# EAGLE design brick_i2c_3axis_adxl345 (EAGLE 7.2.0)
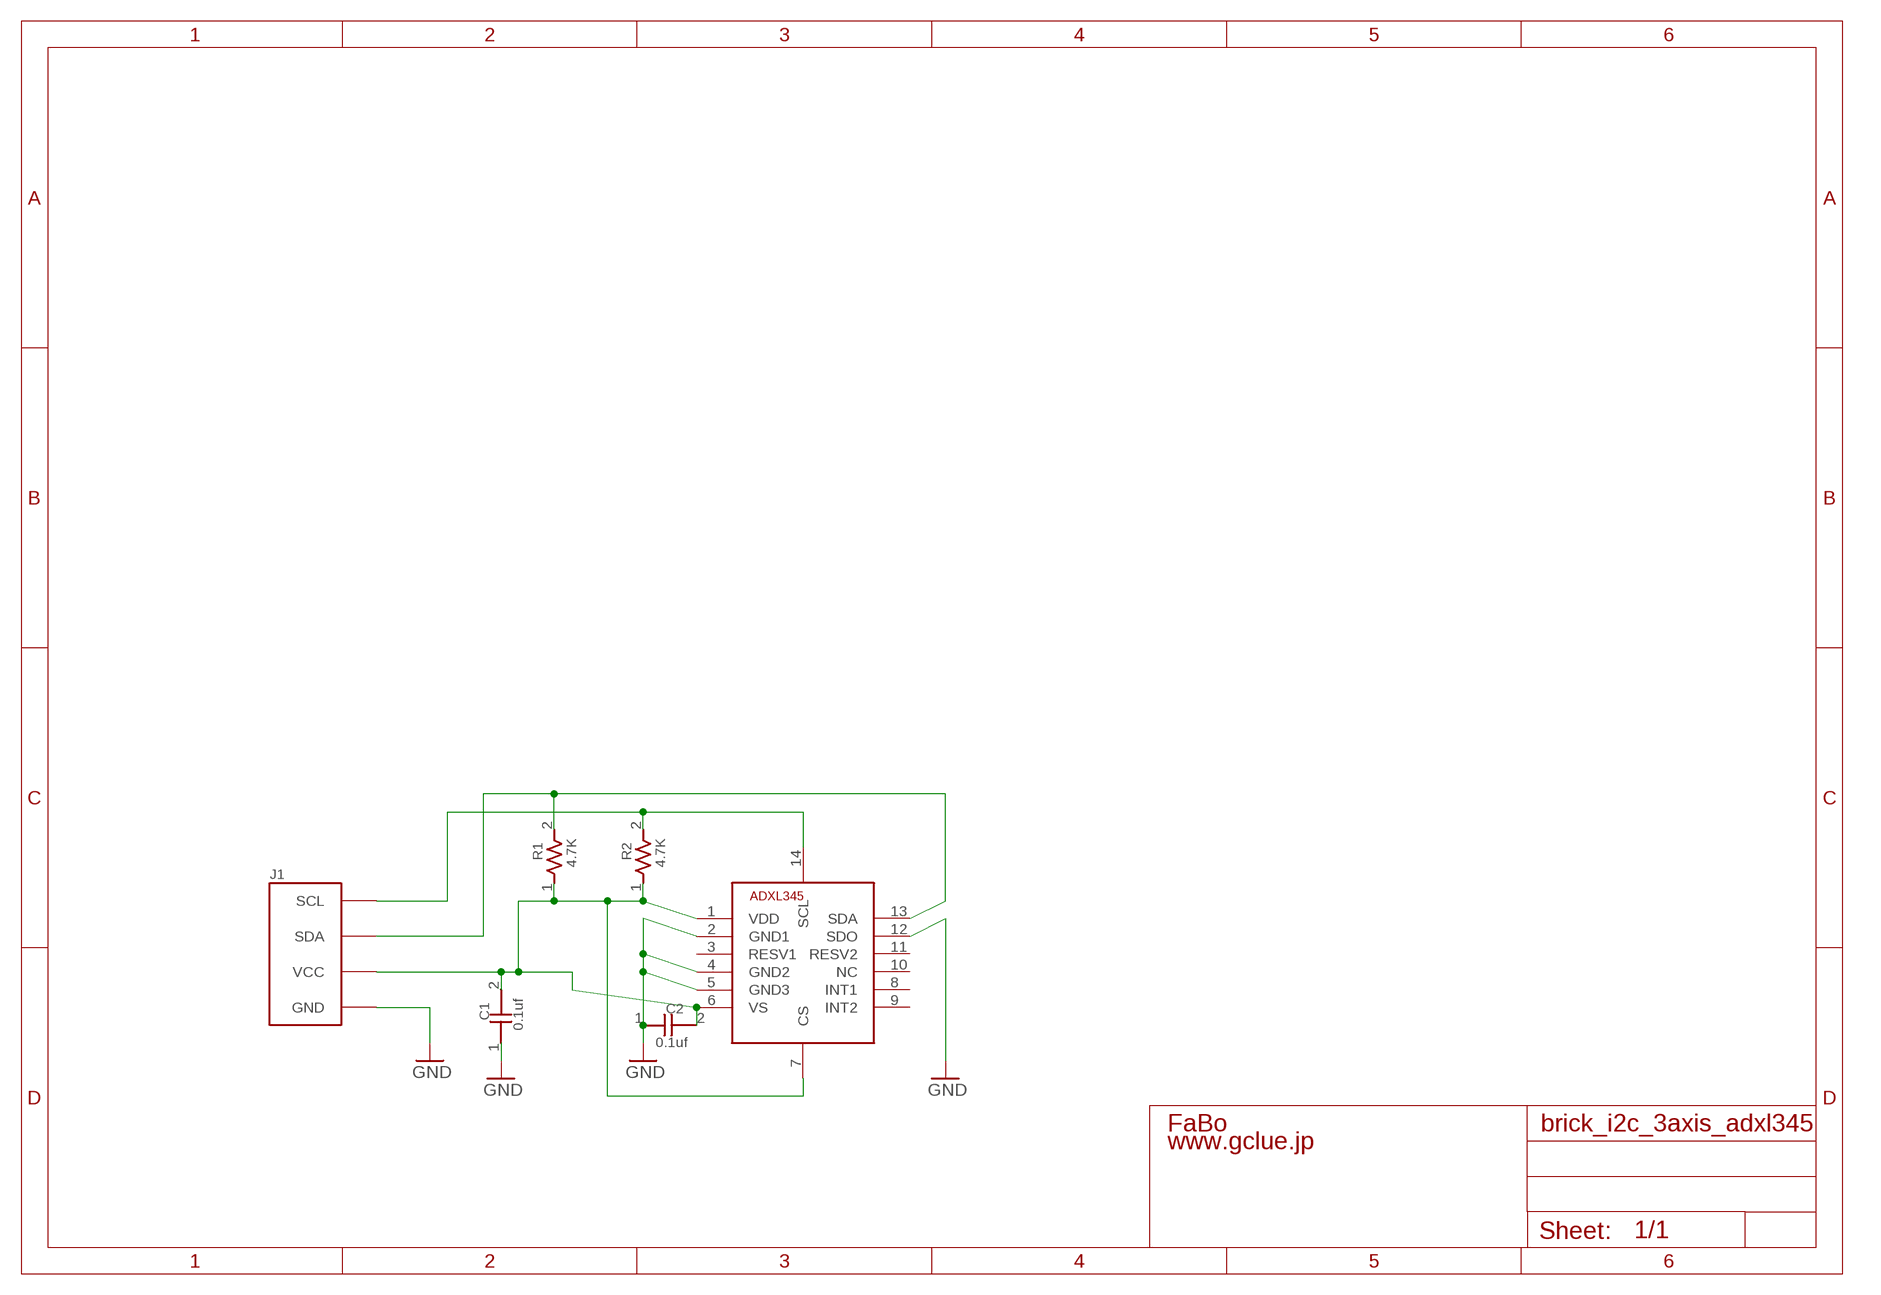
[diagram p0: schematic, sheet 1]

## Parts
C1  0.1uf  CAPACITOR0603  [0603]
C2  0.1uf  CAPACITOR0603  [0603]
J1  BRICK_I2C  [BRICK_I2C]
R1  4.7K  RESISTOR0603  [0603]
R2  4.7K  RESISTOR0603  [0603]
U$2  ANALOGDEVICES-ADXL345  [ANALOGDEVICES-ADXL345]

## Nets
GND: C1.1 C2.1 J1.GND U$2.2(GND1) U$2.4(GND2) U$2.5(GND3) U$2.12(SDO)
N$1: C1.2 C2.2 J1.VCC R1.1 R2.1 U$2.1(VDD) U$2.6(VS) U$2.7(CS)
N$3: J1.SDA R1.2 U$2.13(SDA)
N$4: J1.SCL R2.2 U$2.14(SCL)
Unconnected: U$2.3(RESV1) U$2.8(INT1) U$2.9(INT2) U$2.10(NC) U$2.11(RESV2)

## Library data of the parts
C1 C2 = GClue-Capacitor:CAPACITOR
J1 = gclue:BRICK_I2C: FaBo Brick 4pin(I2C)
R1 R2 = GClue-Resistors:RESISTOR
U$2 = GClue-Mems:ANALOGDEVICES-ADXL345

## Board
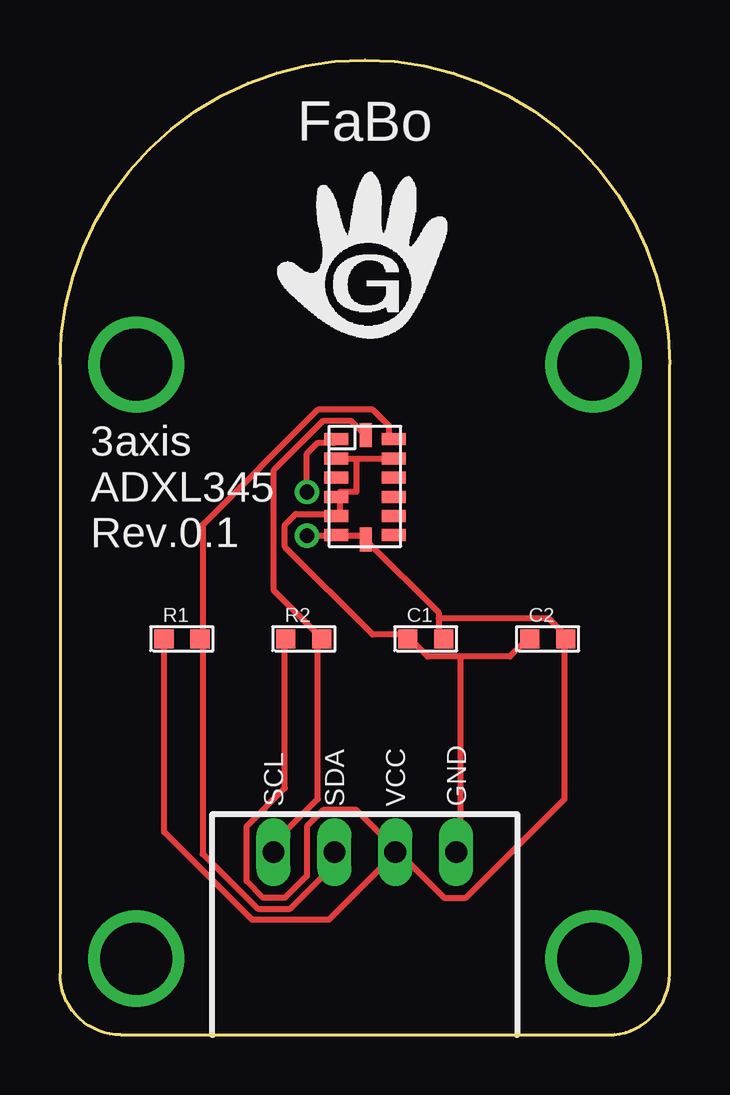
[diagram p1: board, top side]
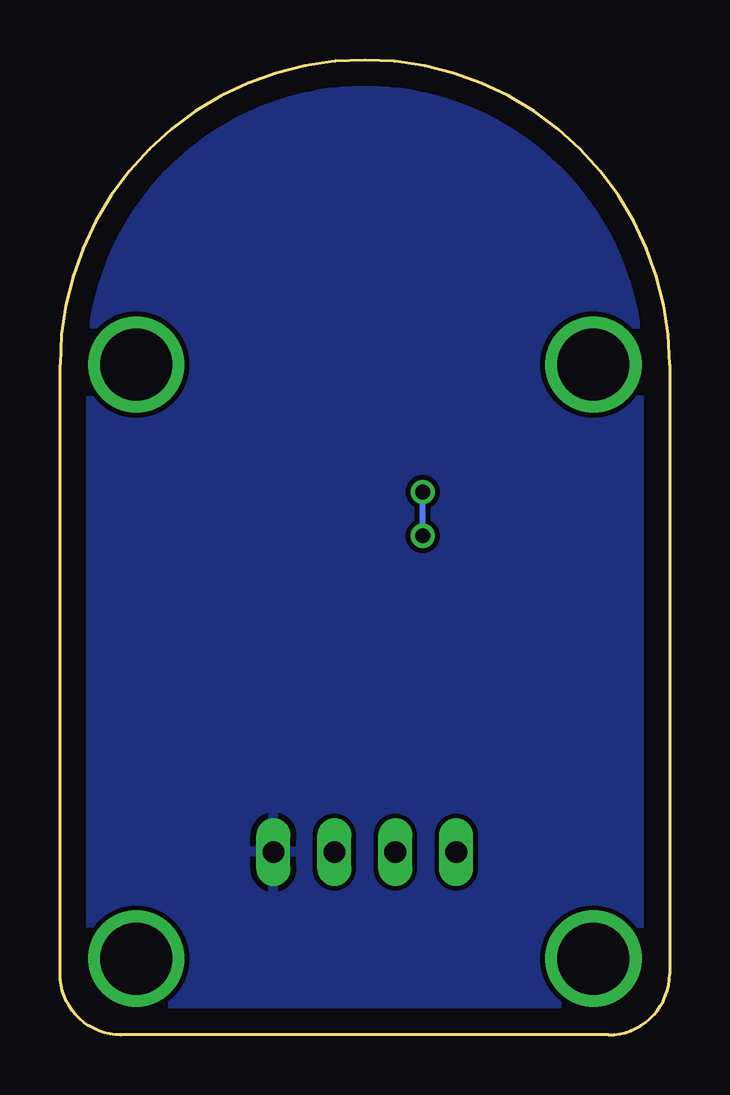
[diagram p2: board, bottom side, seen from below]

Size 25.4 x 40.64 mm. Coordinates in mm from the lower left corner, seen from the top.
Copper layers (1*16): Top 0.035mm / dielectric 1.5mm / Bottom 0.035mm
Design rules "default": minimum track width 10mil, minimum drill 24mil, track to track 8mil, track to pad 8mil, pad to pad 8mil, via to via 8mil, smd to smd 8mil, copper to edge 40mil, drill to drill 8mil, minimum pad ring 10mil, minimum via ring 8mil, stop-mask expansion 4mil, vias tented up to drill 0mil, thermal gap 10mil

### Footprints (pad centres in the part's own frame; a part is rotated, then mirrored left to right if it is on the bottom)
0603 = smd 0.8 x 0.8: 1 -0.75,0; 2 0.75,0
BRICK_I2C = drill 0.9 long: GND 3.81,-12.7; SCL -3.81,-12.7; SDA -1.27,-12.7; VCC 1.27,-12.7 | drill 3 pad 3.81: P$5 -9.525,7.62; P$6 9.525,7.62; P$7 -9.525,-17.145; P$8 9.525,-17.145
ANALOGDEVICES-ADXL345 = smd 1 x 0.5: 1 -1.2,1.97; 2 -1.2,1.17; 3 -1.2,0.37; 4 -1.2,-0.43; 5 -1.2,-1.23; 6 -1.2,-2.03; 8 1.2,-2.03; 9 1.2,-1.23; 10 1.2,-0.43; 11 1.2,0.37; 12 1.2,1.17; 13 1.2,1.97 | smd 0.5 x 1: 7 0.03,-2.2; 14 0.03,2.15

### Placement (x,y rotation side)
C1  15.24,16.51 0 top
C2  20.32,16.51 0 top
J1  12.7,20.32 0 top
R1  5.08,16.51 0 top
R2  10.16,16.51 0 top
U$2  12.7,22.86 0 top

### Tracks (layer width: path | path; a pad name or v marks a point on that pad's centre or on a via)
GND
  Top 0.254: 12.34,24 13.72,24 U$2.12 | 12.34,24 11.66,24 U$2.2 | 12.34,24 12.34,22.63 11.66,22.63 U$2.4 11.66,22.4 11.66,21.72 U$2.5 11.43,21.72 9.83,21.72 9.37,21.26 9.37,20.34 13.03,16.69 14.4,16.69 C1.1 14.63,16.46 15.32,15.77 16.69,15.77 | 16.69,15.77 18.75,15.77 19.43,16.46 C2.1 | 16.69,15.77 16.69,7.77 J1.GND
  pour Bottom: 0,0 25.4,0 25.4,41.91 0,41.91
N$1  (via drill 0.61)
  Top 0.254: 15.77,17.37 15.77,17.6 12.8,20.57 U$2.7 12.57,20.8 11.66,20.8 U$2.6 11.43,20.8 v10.29,20.8 | 15.77,17.37 15.77,16.69 C1.2 | 15.77,17.37 20.34,17.37 21.03,16.69 C2.2 21.03,16.46 21.03,9.83 16.92,5.71 16,5.71 14.17,7.54 J1.VCC | v10.29,22.63 10.29,24.23 10.74,24.69 11.43,24.69 U$2.1 | R1.1 4.34,16.46 4.34,8.46 8,4.8 11.2,4.8 13.95,7.54 J1.VCC | R2.1 9.37,16.46 9.37,10.29 7.77,8.69 7.77,6.4 8.46,5.71 9.37,5.71 10.29,6.63 10.29,8.69 10.97,9.37 12.34,9.37 13.95,7.77 J1.VCC
  Bottom 0.254: v10.29,20.8 v10.29,22.63
N$3
  Top 0.254: U$2.13 13.72,24.92 13.72,25.38 13.03,26.06 10.74,26.06 5.94,21.26 5.94,16.69 R1.2 5.94,16.46 5.94,7.54 8.23,5.26 9.6,5.26 11.43,7.09 J1.SDA
N$4
  Top 0.254: J1.SCL 8.69,7.77 10.74,9.83 10.74,16.46 R2.2 10.74,16.69 8.91,18.52 8.91,23.55 10.97,25.6 12.12,25.6 12.57,25.15 U$2.14

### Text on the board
tPlace: 3axis / ADXL345 / Rev.0.1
